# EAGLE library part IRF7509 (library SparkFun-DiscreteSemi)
Dual N and P Channel MOSFET Dual N/P-Channel 30V 1.25 W 7.8/7.5 nC Hexfet Power Mosfet Surface Mount-MICRO-8. NMOS RDS(ON) 0.11Ω. PMOS RDS(ON) 0.20Ω. Link to datasheet SparkFun Products: SparkFun RedBot Mainboard SparkFun Wake on Shake
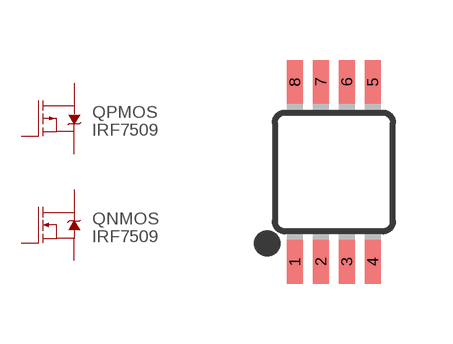
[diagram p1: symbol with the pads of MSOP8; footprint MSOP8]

Designator prefix Q; gates NMOS=LABELED-NMOS PMOS=LABELED-PMOS

## IRF7509 (PROD_ID: TRANS-07913)  [MSOP8]
1  NMOS:S
2  NMOS:G
3  PMOS:S
4  PMOS:G
5  PMOS:D
6  PMOS:D
7  NMOS:D
8  NMOS:D

## Footprint MSOP8 (pad centres in mm)
8M, 8-Lead, 0.118" Wide, Miniature Small Outline Package MSOP 8M-Package doc1097.pdf
smd 0.4 x 1.1: 1 -0.975,-2.25; 2 -0.325,-2.25; 3 0.325,-2.25; 4 0.975,-2.25; 5 0.975,2.25; 6 0.325,2.25; 7 -0.325,2.25; 8 -0.975,2.25

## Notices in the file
Licensing: Creative Commons ShareAlike 4.0 International - https://creativecommons.org/licenses/by-sa/4.0
